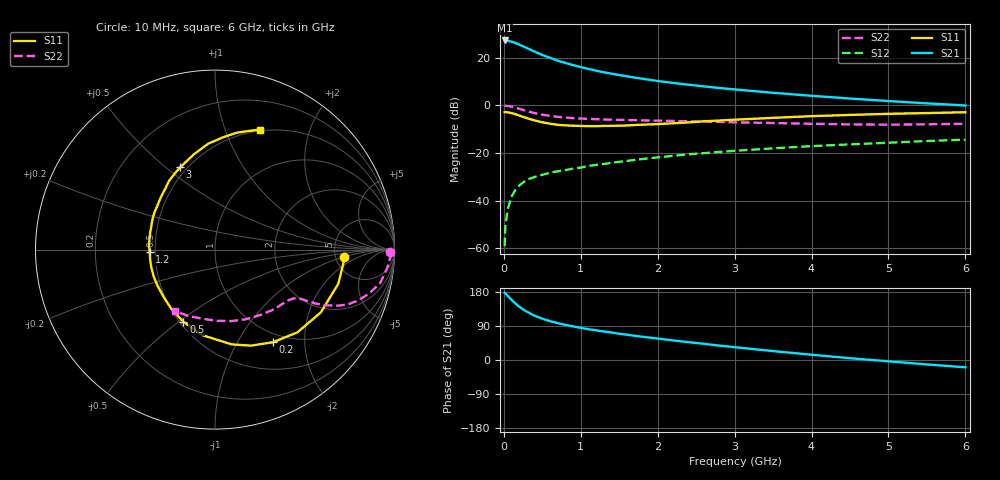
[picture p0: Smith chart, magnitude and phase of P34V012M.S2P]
! SIEMENS Small Signal Semiconductors
! BFP181
! Si NPN RF Bipolar Junction Transistor in SOT143
! VCE = 4 V  IC = 12 mA
! Common Emitter S-Parameters:  March  1996
# GHz  S  MA  R  50
!  f  S11  S21  S12  S22
! GHz  MAG  ANG  MAG  ANG  MAG  ANG  MAG  ANG
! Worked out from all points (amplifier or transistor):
!   36 points, 10 MHz to 6 GHz, reference 50 ohm
!   highest |S21| = 27.2 dB at 10 MHz (marker M1)
!   |S21| within 3 dB of that: start of sweep to 286.5 MHz
!   unconditionally stable (mu >= 1): 1.047 GHz to end of sweep
!   at 250 MHz: K = 0.37, MSG = 28.6 dB, |S12| = -32.4 dB
!   at 1.4 GHz: K = 1.10, MAG = 16.8 dB, |S12| = -24.2 dB
!   at 6 GHz: K = 1.00, MAG = 6.9 dB, |S12| = -14.4 dB
!   S11 on the Smith chart (normalised r, x): 10 MHz: 5.93, -0.98; 200 MHz: 0.87, -1.43; 500 MHz: 0.52, -0.52; 1.2 GHz: 0.47, -0.02; 3 GHz: 0.46, +0.56; 6 GHz: 0.49, +1.33
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0.01  0.7183 -3.2  22.99 177.4  0.0011 87.7  0.9774 -0.9
0.02  0.7191 -6.5  22.95 175.7  0.0029 79.8  0.9787 -2.3
0.05  0.7124 -15.6  22.76 168.9  0.0066 83.1  0.9665 -5.8
0.1  0.6857 -30.6  21.6 158.7  0.0121 74.5  0.9397 -11.3
0.15  0.6507 -45.1  20.4 149.0  0.0167 69.4  0.8932 -15.9
0.2  0.6089 -57.9  18.92 140.7  0.0206 65.2  0.846 -19.6
0.25  0.5716 -69.4  17.29 133.4  0.0239 61.1  0.7991 -22.5
0.3  0.536 -80.1  15.91 127.4  0.0273 57.4  0.7559 -24.4
0.4  0.4818 -98.3  13.4 116.8  0.0313 54.0  0.6852 -26.9
0.5  0.4394 -113.6  11.38 109.0  0.0347 52.0  0.6353 -28.2
0.6  0.4105 -126.3  9.921 102.6  0.0383 51.4  0.5983 -29.0
0.7  0.3891 -137.5  8.641 97.3  0.041 50.3  0.5724 -29.4
0.9  0.3731 -156.0  6.984 88.7  0.0468 50.4  0.5375 -30.4
1.1  0.3654 -171.4  5.814 81.3  0.0532 50.5  0.5173 -31.7
1.2  0.3643 -177.8  5.337 78.3  0.0559 50.8  0.5106 -32.5
1.7  0.3846 155.8  3.814 63.9  0.0712 50.3  0.4865 -37.6
2.2  0.4189 136.4  2.949 51.6  0.0867 48.0  0.4687 -44.3
3  0.4982 112.9  2.154 33.8  0.1105 43.0  0.4389 -57.1
3.5  0.5448 102.3  1.83 23.5  0.1248 39.4  0.4238 -66.5
4.5  0.6274 85.9  1.386 4.7  0.1512 31.5  0.3972 -88.3
5.5  0.6863 74.3  1.097 -11.7  0.1777 24.4  0.398 -111.2
6  0.7149 69.3  0.991 -19.3  0.1903 20.2  0.4102 -122.9
